(* Logix 5000 AddOnInstructionDefinition export AMCI_3204_AOP_Preset; software revision 20.03 *)

ADD_ON_INSTRUCTION AMCI_3204_AOP_Preset   (* revision 1.0, vendor AMCI, ExecuteEnableInFalse *)
VAR_INPUT
   axis_status_bits : INT; {required}
   channel_number : INT; {required}
   Target_Position : DINT; {required}
END_VAR
VAR_IN_OUT
   AMCI_3204_output_data : AM:1756_3204:O:0; {required}
END_VAR
VAR_OUTPUT
   EN : BOOL; {access Read Only, visible}
   ER : BOOL; {access Read Only, visible}
END_VAR
VAR
   command_data_block : DINT[8]; {access None}
END_VAR

ROUTINE EnableInFalse   (* ladder *)
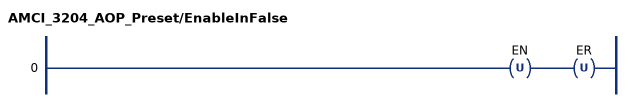
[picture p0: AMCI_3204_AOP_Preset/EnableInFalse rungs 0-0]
   0: OTU(EN)OTU(ER);
END_ROUTINE

ROUTINE Logic   (* ladder *)
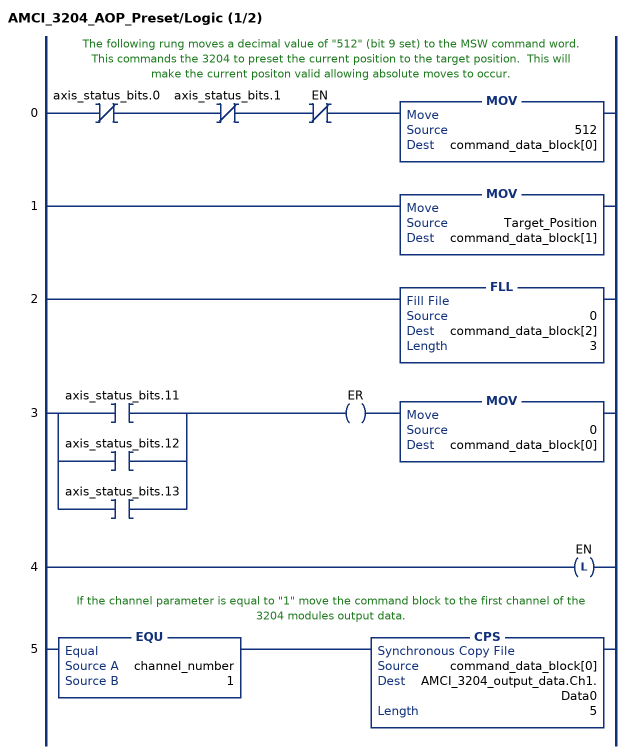
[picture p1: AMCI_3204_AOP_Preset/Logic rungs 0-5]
   // The following rung moves a decimal value of "512" (bit 9 set) to the MSW command word.  This commands the 3204 to preset the current position to the target position.  This will make the current positon valid allowing absolute moves to occur.
   0: XIO(axis_status_bits.0)XIO(axis_status_bits.1)XIO(EN)MOV(512,command_data_block[0]);
   1: MOV(Target_Position,command_data_block[1]);
   2: FLL(0,command_data_block[2],3);
   3: [XIC(axis_status_bits.11) ,XIC(axis_status_bits.12) ,XIC(axis_status_bits.13) ]OTE(ER)MOV(0,command_data_block[0]);
   4: OTL(EN);
   // If the channel parameter is equal to "1" move the command block to the first channel of the 3204 modules output data.
   5: EQU(channel_number,1)CPS(command_data_block[0],AMCI_3204_output_data.Ch1.Data0,5);
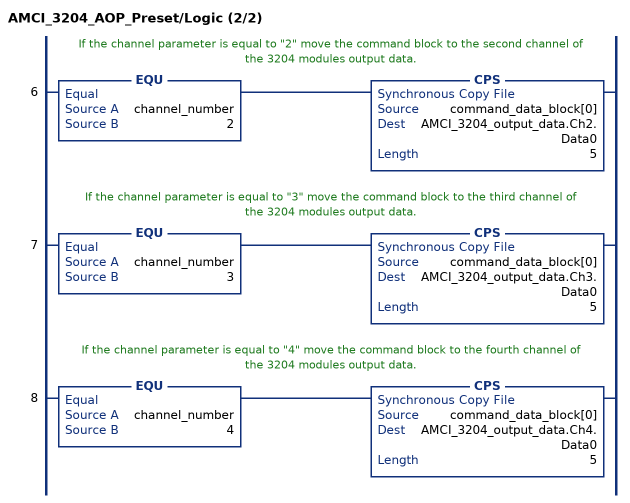
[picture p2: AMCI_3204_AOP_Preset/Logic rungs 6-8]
   // If the channel parameter is equal to "2" move the command block to the second channel of the 3204 modules output data.
   6: EQU(channel_number,2)CPS(command_data_block[0],AMCI_3204_output_data.Ch2.Data0,5);
   // If the channel parameter is equal to "3" move the command block to the third channel of the 3204 modules output data.
   7: EQU(channel_number,3)CPS(command_data_block[0],AMCI_3204_output_data.Ch3.Data0,5);
   // If the channel parameter is equal to "4" move the command block to the fourth channel of the 3204 modules output data.
   8: EQU(channel_number,4)CPS(command_data_block[0],AMCI_3204_output_data.Ch4.Data0,5);
END_ROUTINE
END_ADD_ON_INSTRUCTION
